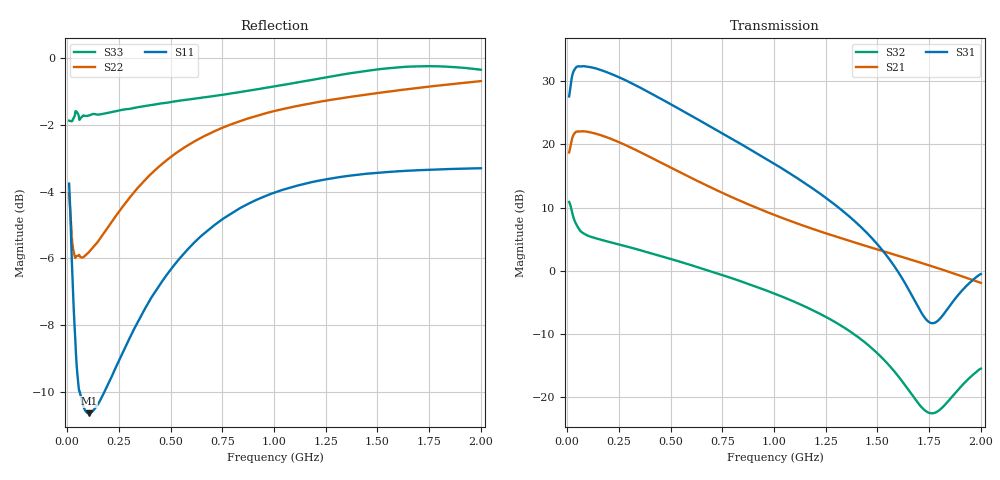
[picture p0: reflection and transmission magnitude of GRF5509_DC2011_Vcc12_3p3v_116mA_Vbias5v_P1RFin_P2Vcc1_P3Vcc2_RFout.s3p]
!Keysight Technologies,N5244B,MY57181157,A.18.40.03
!Date: Wednesday, April 29, 2026 14:30:50
!Correction: S11(C  3-Port  )
!S12(C  3-Port  )
!S13(C  3-Port  )
!S21(C  3-Port  )
!S22(C  3-Port  )
!S23(C  3-Port  )
!S31(C  3-Port  )
!S32(C  3-Port  )
!S33(C  3-Port  )
!S3P File: Measurements: <S11,S12,S13>,
!<S21,S22,S23>,
!<S31,S32,S33>:
# Hz S  dB  R 50
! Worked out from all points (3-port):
!   1991 points, 10 MHz to 2 GHz, reference 50 ohm
!   strongest paths, dB at 10 MHz, 507 MHz, 1.005 GHz, 1.503 GHz, 2 GHz:
!     S31: 27.6, 26.3, 16.9, 4.1, -0.5
!     S21: 18.7, 16.2, 8.8, 3.3, -1.9
!     S32: 10.9, 1.8, -3.6, -13.2, -15.5
!   lowest |S11| = -10.6 dB at 105 MHz (marker M1), VSWR 1.83, Z = 31.1 - j15.1 ohm
!   |S11| at or under -10 dB: 61.27 MHz to 180.7 MHz (119.5 MHz wide, 98.7 % of centre)
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1e7  -3.76 -53.0  -22.21 -33.6  -57.06 -87.2
     18.74 -136.6  -4.05 -77.8  -32.03 -84.0
     27.60 77.4  10.91 -174.5  -1.87 -115.7
3e7  -7.18 -89.6  -26.57 -42.5  -67.13 57.9
     21.44 -161.6  -5.74 -121.8  -43.15 146.6
     31.46 32.0  8.56 161.5  -1.81 -149.5
4.4e7  -8.96 -106.7  -28.65 -42.3  -66.26 -54.4
       22.01 -172.8  -5.94 -136.1  -42.91 -36.6
       32.22 15.9  7.41 157.9  -1.59 -159.4
1.05e8  -10.64 -130.8  -32.31 -30.5  -74.08 -97.4
        21.97 163.2  -5.81 -156.0  -50.95 32.0
        32.27 -17.0  5.50 153.6  -1.72 -170.1
1.72e8  -10.11 -136.5  -33.25 -24.8  -69.92 75.4
        21.37 146.0  -5.30 -160.5  -45.38 44.9
        31.68 -38.9  4.84 146.8  -1.66 -172.6
2.51e8  -9.06 -138.9  -33.72 -22.9  -66.75 83.9
        20.36 129.4  -4.60 -163.1  -42.53 43.5
        30.63 -59.7  4.18 137.7  -1.56 -173.4
4.75e8  -6.55 -144.6  -34.76 -25.1  -61.45 83.6
        16.77 95.2  -3.09 -170.0  -39.70 32.9
        26.84 -105.3  2.13 113.3  -1.34 -173.5
6.71e8  -5.20 -150.3  -35.66 -27.2  -57.75 84.9
        13.57 75.6  -2.30 -175.5  -39.27 28.7
        23.23 -135.1  0.17 94.8  -1.16 -173.3
1.005e9  -4.02 -159.2  -36.95 -28.6  -54.86 85.9
         8.81 54.2  -1.57 177.6  -39.87 30.1
         16.88 -174.9  -3.64 67.0  -0.84 -173.5
2e9  -3.29 -178.0  -39.82 -43.9  -48.16 89.8
     -1.90 10.9  -0.68 156.3  -34.85 70.9
     -0.51 -126.3  -15.48 122.2  -0.34 172.2
